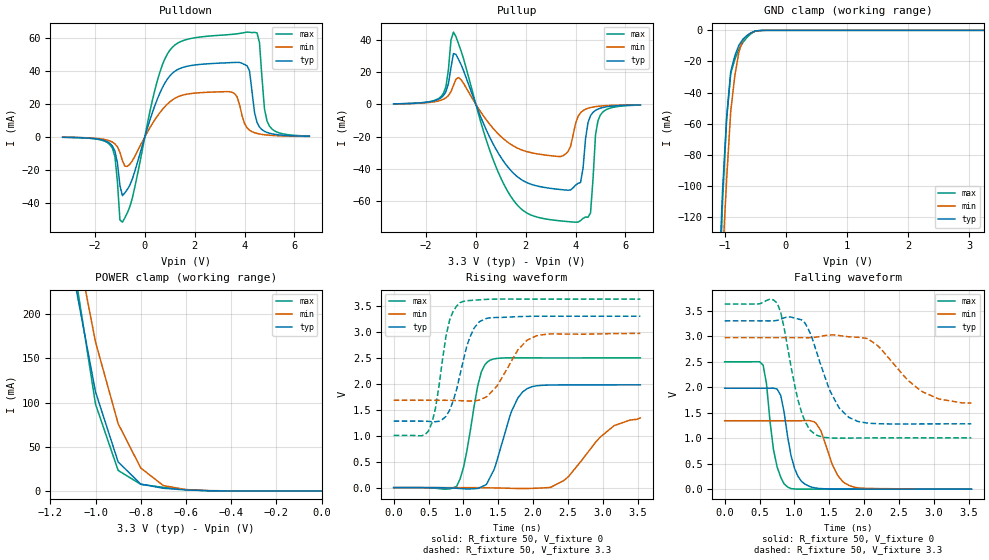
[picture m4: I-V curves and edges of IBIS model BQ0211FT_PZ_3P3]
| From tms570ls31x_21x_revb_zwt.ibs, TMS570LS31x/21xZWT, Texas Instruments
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|   Model Cell BQ0211FT_PZ_3P3
|BQ0211FT_PZ_3P3
[Model]   BQ0211FT_PZ_3P3
Model_type   I/O
Polarity   Non-Inverting
Enable   Active-Low
Vinl =  1.15
Vinh =  1.55
Cref =  15.0001pF
Rref =  101.0000M
Vref =  0V
Vmeas =  1.65
C_comp   1.2p   1.2p   1.2p
[Model Spec]
Vinl   1.15   1.02   1.28
Vinh   1.55   1.45   1.65
[Temperature Range]   25   155   -40
[Voltage Range]   3.3   2.97   3.63
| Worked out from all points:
|   slope of the pulldown table from 0 to 0.495 V, typ, clamps not added: 22 ohm
|   slope of the pullup table from 0 to 0.495 V, typ, clamps not added: 26.9 ohm
|   GND clamp passes 1 mA (typ) near -0.53 V on its own axis
|   POWER clamp passes 1 mA (typ) near -0.59 V on its own axis
|   rising waveform, R_fixture 50, V_fixture 0: 20-80 % time 278ps typ, 513ps min, 195ps max; typ from 0 V to 1.98 V
|   rising waveform, R_fixture 50, V_fixture 3.3: 20-80 % time 239ps typ, 354ps min, 182ps max; typ from 1.28 V to 3.3 V
|   falling waveform, R_fixture 50, V_fixture 0: 20-80 % time 164ps typ, 225ps min, 138ps max; typ from 1.98 V to 0 V
|   falling waveform, R_fixture 50, V_fixture 3.3: 20-80 % time 335ps typ, 536ps min, 238ps max; typ from 3.3 V to 1.28 V
[POWER_clamp]
|   voltage   I(typ)   I(min)   I(max)
-3.3V     4.054A     4.63A      4.887A
-1.1V     248.3mA    301mA      262.7mA
-1.067V   202.9mA    256.9mA    207.9mA
-1.033V   157.5mA    212.7mA    153.1mA
-1V       112.1mA    168.6mA    98.29mA
-900mV    32.88mA    76.23mA    23.22mA
-800mV    7.705mA    25.95mA    7.475mA
-700mV    3.033mA    6.039mA    3.99mA
-600mV    1.087mA    1.528mA    1.425mA
-500mV    187uA      368.9uA    203.4uA
0V        443pA      6.158nA    417pA
[Pulldown]
|   voltage   I(typ)   I(min)   I(max)
-3.3V     -289uA     -253.9uA   -287.1uA
-1.4V     -4mA       -2.489mA   -4.76mA
-1.2V     -8.69mA    -4.261mA   -12.05mA
-1V       -29.49mA   -9.376mA   -50.19mA
-900mV    -35.6mA    -14.42mA   -51.59mA
1V        36.78mA    21.07mA    52.28mA
3.5V      44.86mA    26.91mA    61.93mA
4.1V      42.98mA    5.455mA    63.29mA
4.6V      5.887mA    1.718mA    56.92mA
4.8V      3.323mA    1.257mA    16.92mA
5V        2.171mA    957.9uA    6.458mA
6.6V      331.3uA    239.5uA    466.8uA
[Pullup]
|   voltage   I(typ)   I(min)   I(max)
-3.3V     325.3uA    297.6uA    301.6uA
-1.4V     4.042mA    2.556mA    4.795mA
-1.2V     7.932mA    4.062mA    11.12mA
-900mV    31.45mA    11.76mA    44.76mA
1.4V      -40.91mA   -24.77mA   -56.99mA
3.4V      -52.76mA   -32.29mA   -72.18mA
4V        -50.08mA   -11.8mA    -72.98mA
4.2V      -48.37mA   -5.201mA   -71.98mA
4.6V      -7.019mA   -1.989mA   -67.23mA
4.8V      -3.708mA   -1.414mA   -19.03mA
5V        -2.349mA   -1.055mA   -6.475mA
6.6V      -340.9uA   -258.1uA   -448.7uA
[GND_clamp]
|   voltage   I(typ)   I(min)   I(max)
-3.3V     -3.25A     -2.875A    -4.945A
-1.1V     -166.9mA   -205mA     -187mA
-1.033V   -102.7mA   -146.7mA   -110.1mA
-966.7mV  -55.96mA   -95.69mA   -57.01mA
-900mV    -26.55mA   -52.03mA   -27.79mA
-833.3mV  -16.49mA   -29.28mA   -18.76mA
-766.7mV  -9.537mA   -13.91mA   -12.06mA
-700mV    -5.687mA   -5.923mA   -7.702mA
-566.7mV  -1.566mA   -1.63mA    -2.054mA
-500mV    -402.1uA   -594uA     -459.6uA
-366.7mV  -18.7uA    -59.22uA   -17.4uA
3.233V    423.5pA    4.09uA     323pA
[Ramp]
| variable   typ   min   max
dV/dt_f   1.260456/0.3438705n  0.8122496/0.5595305n   1.63828/0.2454093n
dV/dt_r   1.203486/0.2797523n  0.8165939/0.5189431n   1.518027/0.1974225n
R_load = 50
[Rising Waveform]
R_fixture = 50
V_fixture = 0
V_fixture_min = 0
V_fixture_max = 0
|   time   V(typ)   V(min)   V(max)
0s        -6.166uV   -3.049uV   -3.574uV
904ps     -12.7mV    195.5uV    26.05mV
1.004ns   -22.19mV   252uV      398.2mV
1.256ns   11.7mV     -1.83mV    2.219V
1.384ns   198.8mV    -4.337mV   2.455V
1.696ns   1.484V     -13.98mV   2.498V
1.916ns   1.907V     -16.84mV   2.498V
2.444ns   1.978V     139.5mV    2.497V
3.164ns   1.978V     1.193V     2.497V
3.54ns    1.979V     1.342V     2.497V
[Rising Waveform]
R_fixture = 50
V_fixture = 3.3
V_fixture_min = 2.97
V_fixture_max = 3.63
|   time   V(typ)   V(min)   V(max)
0s        1.281V     1.682V     1.005V
500ps     1.275V     1.682V     1.092V
600ps     1.269V     1.682V     1.528V
804ps     1.493V     1.68V      3.232V
952ps     2.173V     1.674V     3.563V
1.152ns   3.067V     1.67V      3.608V
1.332ns   3.257V     1.749V     3.625V
1.784ns   3.292V     2.654V     3.63V
2.048ns   3.3V       2.922V     3.63V
3.54ns    3.3V       2.969V     3.63V
[Falling Waveform]
R_fixture = 50
V_fixture = 0
V_fixture_min = 0
V_fixture_max = 0
|   time   V(typ)   V(min)   V(max)
0s        1.979V     1.342V     2.498V
552ps     1.979V     1.342V     2.429V
700ps     1.981V     1.342V     774.6mV
804ps     1.838V     1.342V     232.9mV
904ps     1.021V     1.342V     41.26mV
1.052ns   251.1mV    1.341V     249.1uV
1.256ns   35.11mV    1.331V     658.1uV
1.616ns   2.885mV    282.3mV    445.4uV
1.784ns   1.498mV    72.85mV    465.9uV
3.54ns    277.9uV    525.7uV    20.8uV
[Falling Waveform]
R_fixture = 50
V_fixture = 3.3
V_fixture_min = 2.97
V_fixture_max = 3.63
|   time   V(typ)   V(min)   V(max)
0s        3.3V       2.97V      3.63V
752ps     3.309V     2.97V      3.649V
804ps     3.332V     2.97V      3.466V
1.104ns   3.319V     2.97V      1.503V
1.308ns   2.734V     2.98V      1.063V
1.512ns   1.925V     3.023V     1.006V
1.784ns   1.405V     2.988V     1.002V
2.18ns    1.285V     2.831V     1.005V
2.84ns    1.28V      1.908V     1.006V
3.54ns    1.281V     1.69V      1.006V
